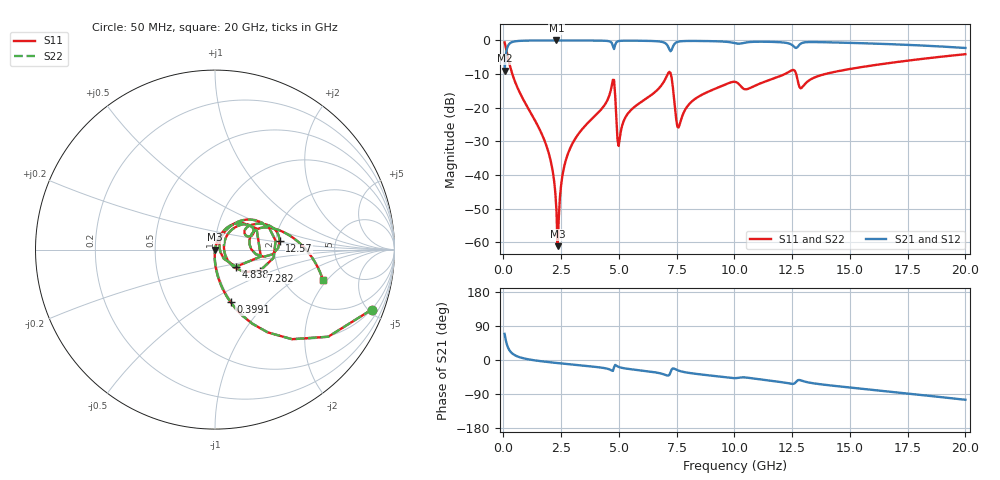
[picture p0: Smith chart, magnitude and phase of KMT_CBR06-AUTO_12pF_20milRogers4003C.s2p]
! Data measured by Modelithics Inc. support@modelithics.com 813-866-6335
! KEMET CBR06-AUTO 12pF, Pad Width= 0.851mm, Pad Length= 0.64mm, Pad Gap= 0.62mm, 20mil Rogers 4003C substrate Data, January 2022
# hz S ma R 50
! 2 Port Network Data from SP1.SP block
! freq  magS11  angS11  magS21  angS21  magS12  angS12  magS22  angS22
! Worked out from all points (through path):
!   401 points, 50 MHz to 20 GHz, reference 50 ohm
!   highest |S21| = -0.01 dB at 2.294 GHz (marker M1); lowest = -9.0 dB at 50 MHz (marker M2)
!   group delay of S21, straight-line fit = 15.3 ps
!   lowest |S11| = -61.2 dB at 2.344 GHz (marker M3), VSWR 1.00, Z = 50.1 - j0.0482 ohm
!   |S11| at or under -10 dB: 384.9 MHz to 7.114 GHz (6.729 GHz wide, 179 % of centre); 7.244 GHz to 12.18 GHz (4.938 GHz wide, 50.8 % of centre); 12.67 GHz to 13.92 GHz (1.25 GHz wide, 9.4 % of centre)
!   |S22| runs from -61.2 to -0.6 dB; largest |S21 - S12| = 0
!   S11 on the Smith chart (normalised r, x): 50 MHz: 0.99, -5.22; 399.1 MHz: 0.99, -0.64; 4.838 GHz: 1.24, -0.24; 7.282 GHz: 1.61, -0.41; 12.57 GHz: 2.11, +0.23; 20 GHz: 3.25, -1.80
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5e7  0.9346 -21.0  0.3553 69.0  0.3553 69.0  0.9346 -21.0
3.99125e8  0.3051 -73.5  0.9519 16.4  0.9519 16.4  0.3051 -73.5
1.895375e9  0.02502 -93.5  0.9989 -5.1  0.9989 -5.1  0.02502 -93.5
2.14475e9  0.01074 -92.8  0.9991 -6.8  0.9991 -6.8  0.01074 -92.8
2.294375e9  0.002989 -82.6  0.9991 -7.8  0.9991 -7.8  0.002989 -82.6
2.34425e9  0.0008743 -33.4  0.9991 -8.1  0.9991 -8.1  0.0008743 -33.4
2.693375e9  0.01624 76.7  0.9989 -10.3  0.9989 -10.3  0.01624 76.7
3.391625e9  0.0472 74.2  0.9977 -14.5  0.9977 -14.5  0.0472 74.2
4.688375e9  0.2113 45.4  0.9184 -27.9  0.9184 -27.9  0.2113 45.4
4.838e9  0.1503 -39.5  0.8632 -12.9  0.8632 -12.9  0.1503 -39.5
5.0375e9  0.03579 46.7  0.9847 -19.3  0.9847 -19.3  0.03579 46.7
5.4365e9  0.08586 63.5  0.9919 -23.7  0.9919 -23.7  0.08586 63.5
6.73325e9  0.1946 51.4  0.9666 -34.4  0.9666 -34.4  0.1946 51.4
7.281875e9  0.2774 -24.9  0.7223 -25.1  0.7223 -25.1  0.2774 -24.9
7.581125e9  0.05087 12.3  0.9604 -28.0  0.9604 -28.0  0.05087 12.3
8.279375e9  0.1339 50.4  0.9825 -36.1  0.9825 -36.1  0.1339 50.4
1.0025e10  0.2424 27.8  0.9115 -47.9  0.9115 -47.9  0.2424 27.8
1.256862e10  0.3638 7.5  0.8158 -62.7  0.8158 -62.7  0.3638 7.5
1.286788e10  0.1944 8.8  0.8943 -53.6  0.8943 -53.6  0.1944 8.8
1.336662e10  0.2712 25.7  0.9464 -61.0  0.9464 -61.0  0.2712 25.7
1.670825e10  0.4613 5.9  0.8811 -83.5  0.8811 -83.5  0.4613 5.9
2e10  0.6246 -15.7  0.7721 -105.0  0.7721 -105.0  0.6246 -15.7
